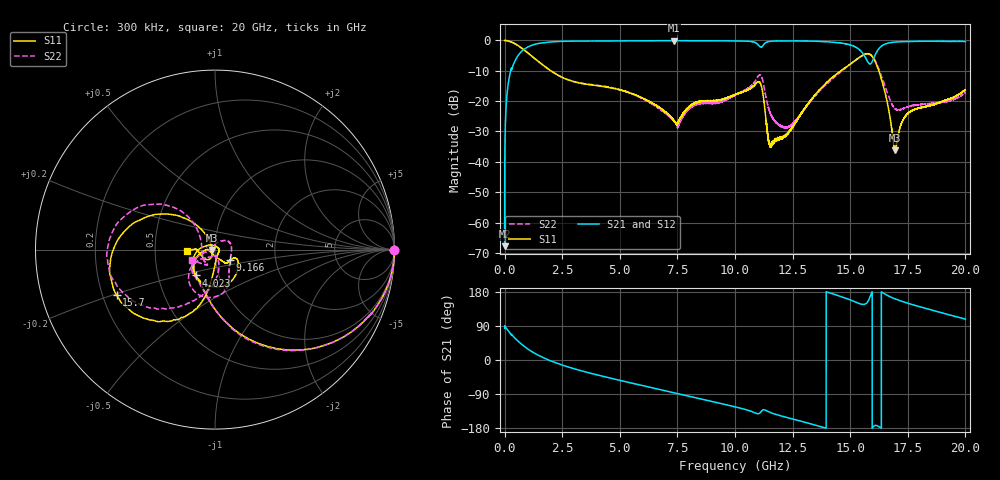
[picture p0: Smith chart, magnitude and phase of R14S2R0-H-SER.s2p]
!{R14S2R0}
!Johanson Technology Inc.
!www.johansontechnology.com
!Test Board Conditions:
!Substrate Type  RO4350B
!Substrate Thickness  20 mil
!Substrate Dk  3.66
!TL Type: GCPW
!TL Trace Width  36 mil
!TL Gap  12 mil
!Electrode orientation  Horizontal
!DUT TOPOLOGY	SERIES
!Mounting Pad LxW  26x36 mil
! Created Wed Nov 25 17:33:21 2020
! 2 Port Network Data from SP1.SP block
! freq  magS11  angS11  magS21  angS21  magS12  angS12  magS22  angS22
# khz S ma R 50
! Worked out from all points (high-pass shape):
!   20001 points, 300 kHz to 20 GHz, reference 50 ohm
!   highest |S21| = -0.05 dB at 7.358 GHz (marker M1); lowest = -67.8 dB at 300 kHz (marker M2)
!   |S21| within 3 dB of the highest: 821.2 MHz to 15.4 GHz (14.58 GHz wide, 180 % of centre); 16.21 GHz to end of sweep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
!   lowest |S11| = -36.2 dB at 16.95 GHz (marker M3), VSWR 1.03, Z = 48.5 - j0.259 ohm
!   |S11| at or under -10 dB: 2.01 GHz to 14.6 GHz (12.59 GHz wide, 152 % of centre); 16.24 GHz to end of sweep
!   |S22| runs from -28.9 to 0.0 dB; largest |S21 - S12| = 0.016
!   S11 on the Smith chart (normalised r, x): 300 kHz: open; 4.023 GHz: 0.78, -0.23; 9.166 GHz: 1.17, -0.14; 15.7 GHz: 0.26, -0.21; 20 GHz: 0.73, -0.01
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300  0.997 -0.1  0.0004079 83.3  0.0004142 87.8  0.9952 -0.2
101300  0.9918 -8.3  0.1261 81.6  0.1265 81.5  0.9915 -8.3
133300  0.9859 -10.9  0.1649 79.0  0.1657 79.0  0.985 -10.9
494300  0.8634 -34.4  0.4968 55.1  0.4977 55.1  0.8623 -34.5
1548300  0.4261 -79.6  0.9003 10.1  0.9007 10.1  0.4263 -79.8
3334300  0.1962 -117.2  0.9763 -28.6  0.9765 -28.5  0.1979 -119.2
4023300  0.1797 -126.8  0.9798 -39.4  0.9793 -39.4  0.1824 -131.2
6667300  0.08084 -167.6  0.9912 -77.0  0.99 -76.9  0.07743 -162.2
7358300  0.04743 -179.0  0.9938 -86.6  0.9928 -86.6  0.04653 -164.6
9166300  0.1012 -36.1  0.986 -111.7  0.9882 -111.7  0.09208 -10.5
1.00003e7  0.1284 -22.7  0.9811 -123.6  0.9798 -123.6  0.1262 -50.3
1.10723e7  0.2055 -101.4  0.797 -140.3  0.7987 -140.2  0.2695 -99.2
1.15623e7  0.01917 49.7  0.9687 -139.3  0.9703 -139.3  0.05991 -133.8
1.23123e7  0.03013 -59.3  0.9825 -152.7  0.9837 -152.6  0.03761 -88.6
1.33343e7  0.1088 -92.5  0.9735 -169.3  0.9751 -169.2  0.1053 -78.6
1.48793e7  0.3775 -111.0  0.8678 161.5  0.8679 161.1  0.3742 -122.2
1.57023e7  0.6039 -155.0  0.4911 149.2  0.4922 149.0  0.5993 -168.8
1.61323e7  0.4095 152.5  0.6272 -172.7  0.6296 -172.5  0.4245 143.6
1.66673e7  0.07308 120.5  0.9085 168.8  0.9062 169.1  0.1209 136.8
1.69493e7  0.01541 -170.0  0.9401 161.4  0.9402 161.5  0.07459 167.8
1.75383e7  0.06428 -121.5  0.9619 149.2  0.9612 149.1  0.08136 -145.3
2e7  0.1536 -177.1  0.9618 107.9  0.9612 108.0  0.1395 -156.8
